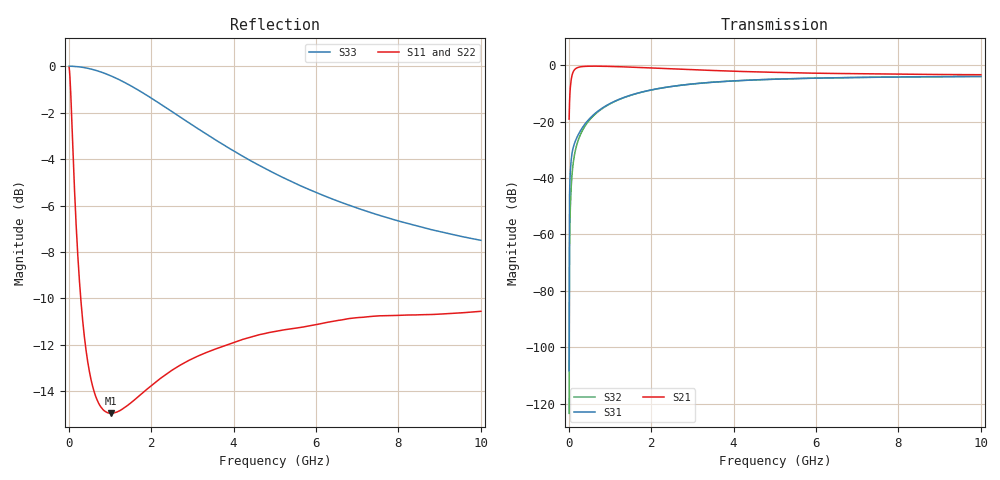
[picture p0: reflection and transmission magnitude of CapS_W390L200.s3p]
! Created Fri Sep 09 14:51:58 2011
# ghz S ma R 50
! 3 Port Network Data from SP1.SP block
! freq  magS11  angS11  magS12  angS12  magS13  angS13
!  magS21  angS21
!  magS22  angS22  magS23  angS23
!  magS31  angS31  magS32  angS32
!  magS33  angS33
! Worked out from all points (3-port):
!   1000 points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, 10 MHz to 10 GHz, reference 50 ohm
!   strongest paths, dB at 10 MHz, 2.51 GHz, 5.01 GHz, 7.51 GHz, 10 GHz:
!     S21: -19.1, -1.2, -2.5, -3.0, -3.3
!     S31: -108.4, -7.4, -4.9, -4.2, -3.9
!     S32: -123.5, -7.4, -4.9, -4.2, -3.9
!   lowest |S11| = -14.9 dB at 1.03 GHz (marker M1), VSWR 1.44, Z = 43.3 - j15.5 ohm
!   |S11| at or under -10 dB: 292.1 MHz to end of sweep
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0.01  0.9937 -6.4  0.1115 83.6  3.804e-06 -3.7
      0.1115 83.6  0.9937 -6.4  6.717e-07 158.3
      3.804e-06 -3.7  6.717e-07 158.3  1 -0.0
0.07  0.7877 -39.6  0.615 51.2  0.02426 72.3
      0.615 51.2  0.7881 -38.0  0.009095 136.5
      0.02426 72.3  0.009095 136.5  0.9996 -1.7
0.09  0.7066 -47.2  0.7064 43.9  0.03019 70.1
      0.7064 43.9  0.7071 -45.0  0.01392 129.8
      0.03019 70.1  0.01392 129.8  0.9994 -2.2
0.12  0.6019 -55.8  0.797 35.6  0.03719 68.7
      0.797 35.6  0.6028 -53.0  0.02118 121.9
      0.03719 68.7  0.02118 121.9  0.9991 -3.0
0.2  0.4216 -69.8  0.9045 22.5  0.0529 69.1
     0.9045 22.5  0.4231 -65.2  0.04002 108.7
     0.0529 69.1  0.04002 108.7  0.9978 -5.0
0.5  0.2206 -89.1  0.9676 6.8  0.1125 71.5
     0.9676 6.8  0.2239 -79.9  0.1065 90.1
     0.1125 71.5  0.1065 90.1  0.9879 -12.5
1.03  0.1789 -103.8  0.9573 -1.4  0.2157 66.6
      0.9573 -1.4  0.1826 -92.8  0.213 75.9
      0.2157 66.6  0.213 75.9  0.9525 -25.1
2.54  0.2225 -129.1  0.8672 -9.7  0.4276 48.1
      0.8672 -9.7  0.2242 -121.9  0.4271 51.9
      0.4276 48.1  0.4271 51.9  0.7947 -55.4
5.01  0.2684 -149.6  0.7528 -11.4  0.5701 30.0
      0.7528 -11.4  0.2684 -145.5  0.5696 31.9
      0.5701 30.0  0.5696 31.9  0.5869 -87.8
10  0.2967 -166.3  0.6833 -8.7  0.637 15.8
    0.6833 -8.7  0.2965 -164.2  0.6371 16.8
    0.637 15.8  0.6371 16.8  0.4218 -121.8
